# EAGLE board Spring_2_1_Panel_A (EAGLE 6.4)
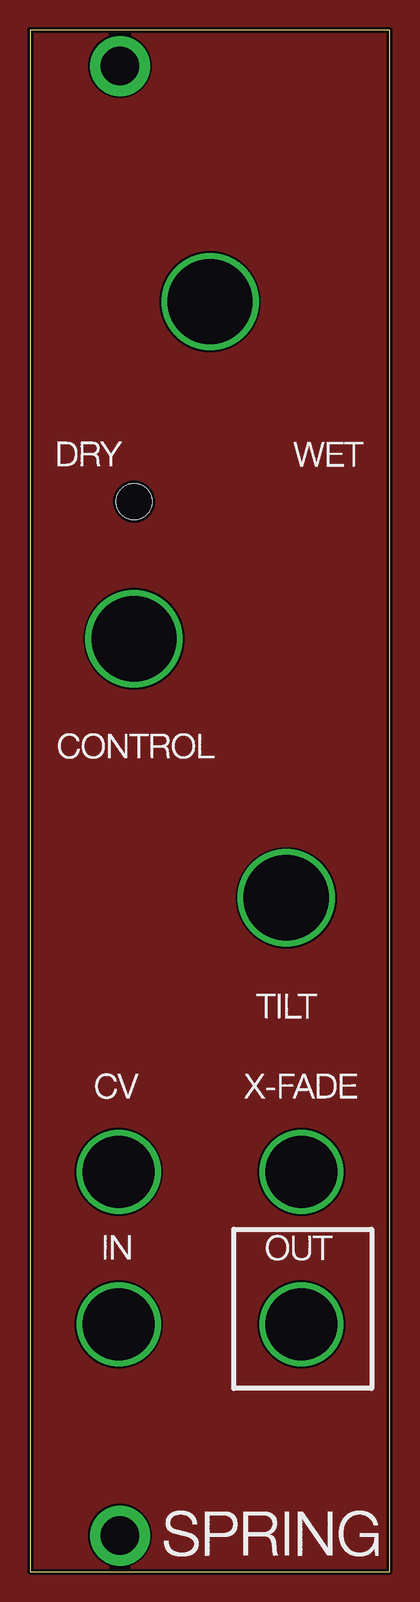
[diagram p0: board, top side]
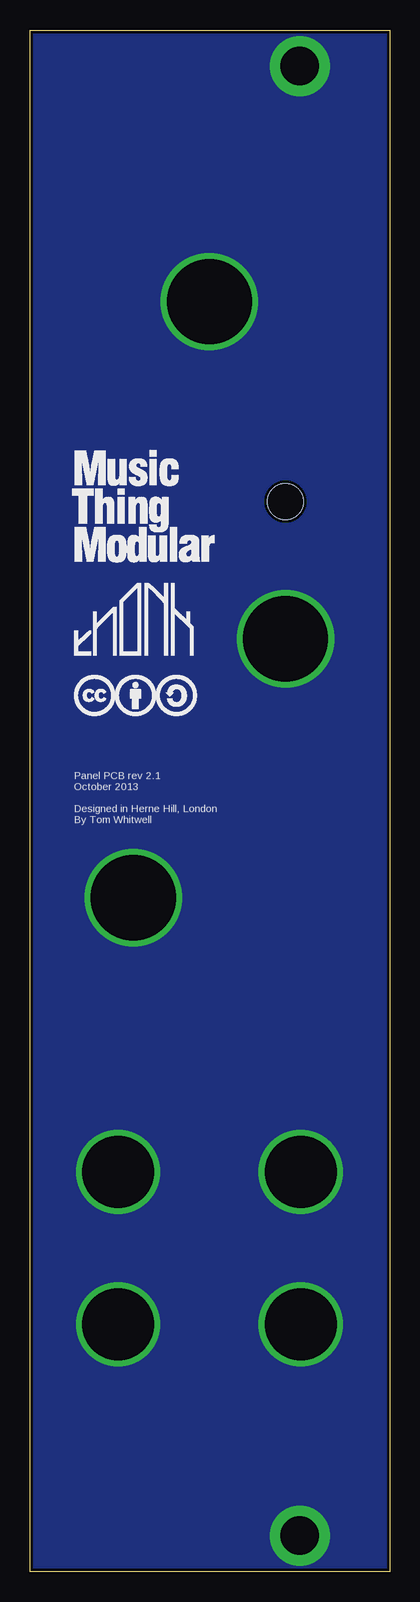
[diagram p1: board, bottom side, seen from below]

Size 30 x 128.5 mm. Coordinates in mm from the lower left corner, seen from the top.
Outline: 0,0 30,0 30,128.5 0,128.5 0,0
Copper layers (1*2*15*16): Top 0.035mm / dielectric 0.2mm / Route2 0.0175mm / dielectric 1.1mm / Route15 0.0175mm / dielectric 0.2mm / Bottom 0.035mm
Design rules "SeeedStudio_DRU_no_angle_20130527": minimum track width 6mil, minimum drill 12mil, track to track 6mil, track to pad 6mil, pad to pad 6mil, via to via 6mil, smd to smd 0mil, copper to edge 10mil, drill to drill 10mil, minimum pad ring 6mil, minimum via ring 6mil, stop-mask expansion 2mil, vias tented up to drill 25mil, thermal gap 10mil
Holes 3 mm at 8.68,89.18

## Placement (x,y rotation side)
U$1  [MTM_1CM_KEEPOUT]  17.44,118.48 0 top
U$2  [THONK_1CM_SCREENPRINT]  26.29,76.37 0 bottom
U$3  [CC_1CM_SCREENPRINT]  26.31,71.32 0 bottom
U$4  [MTM_1CM]  26.55,83.66 0 bottom

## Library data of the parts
U$1-U$4 = TW_logos

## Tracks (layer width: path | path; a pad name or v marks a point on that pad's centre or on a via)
GND  (via drill 3.2 pad 5, 6, 7.1)
  other vias: 7.5,3 7.5,125.5 22.65,33.3 7.41,33.3 22.65,20.6 7.41,20.6 21.38,56.16 8.68,77.75 15.03,105.85
  pour Bottom: -2.5,132 34.5,132 35.5,-5.5 -2.5,-4
N$2
  pour Top: -8.59,137.48 41.88,137.48 41.88,134.05 41.88,-12.37 -11.67,-12.37 -11.67,134.39

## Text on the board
bPlace: Panel PCB rev 2.1 / October 2013 / / Designed in Herne Hill, London / By Tom Whitwell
